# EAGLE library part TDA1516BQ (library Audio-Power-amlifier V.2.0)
radio power amplifier 24 W BTL or 2 x 12 watt stereo car Source: TDA1516BQ_1.pdf
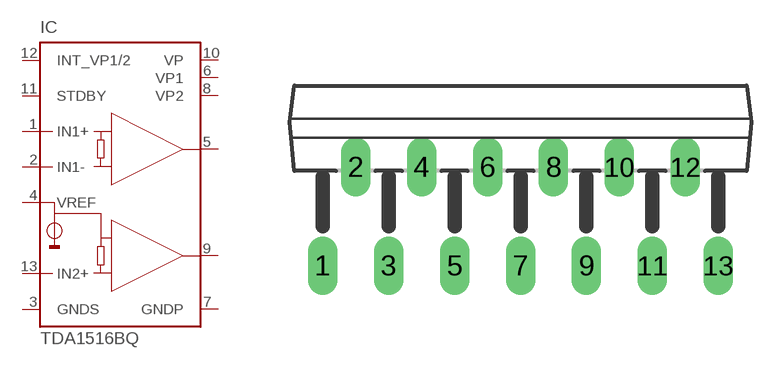
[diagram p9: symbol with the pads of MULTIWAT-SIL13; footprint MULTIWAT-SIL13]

Designator prefix IC

## TDA1516BQ  [MULTIWAT-SIL13]
1  IN1+  in
2  IN1-  in
3  GNDS  pwr
4  VREF  pas
5  OUT1  out
6  VP1  pwr
7  GNDP  pwr
8  VP2  pwr
9  OUT2  out
10  VP  in
11  STDBY  in
12  INT_VP1/2  pas
13  IN2+  in

## Footprint MULTIWAT-SIL13 (pad centres in mm)
DBS13P plastic DIL-bent-SIL power package 13 leads (lead length 12 mm) SOT141-6 Source: TDA1516BQ_1.pdf
drill 1 pad 1.5 long: 1 -10.2,-5.08; 2 -8.5,0; 3 -6.8,-5.08; 4 -5.1,0; 5 -3.4,-5.08; 6 -1.7,0; 7 0,-5.08; 8 1.7,0; 9 3.4,-5.08; 10 5.1,0; 11 6.8,-5.08; 12 8.5,0; 13 10.2,-5.08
